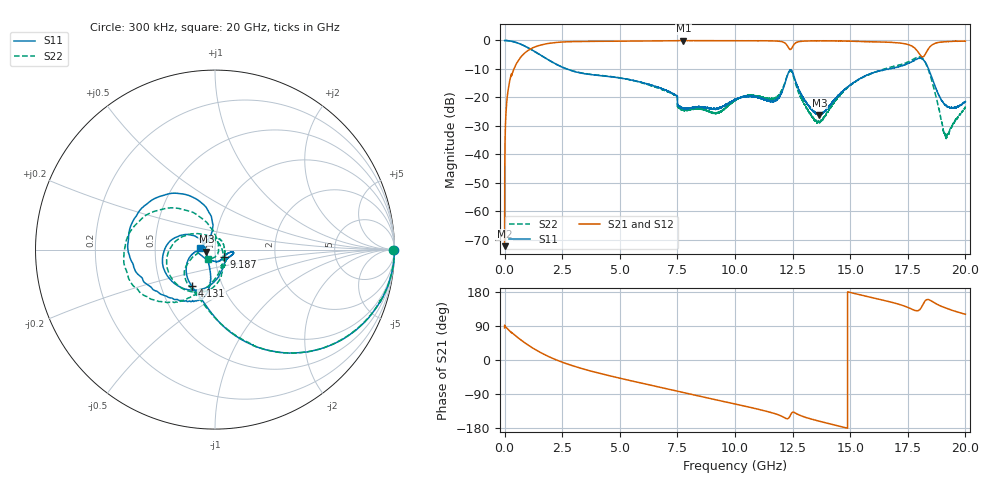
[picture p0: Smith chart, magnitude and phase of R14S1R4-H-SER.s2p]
!{R14S1R4}
!Johanson Technology Inc.
!www.johansontechnology.com
!Test Board Conditions:
!Substrate Type  RO4350B
!Substrate Thickness  20 mil
!Substrate Dk  3.66
!TL Type: GCPW
!TL Trace Width  36 mil
!TL Gap  12 mil
!Electrode orientation  Horizontal
!DUT TOPOLOGY	SERIES
!Mounting Pad LxW  26x36 mil
! Created Wed Nov 25 17:33:21 2020
! 2 Port Network Data from SP1.SP block
! freq  magS11  angS11  magS21  angS21  magS12  angS12  magS22  angS22
# khz S ma R 50
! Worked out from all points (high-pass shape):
!   20001 points, 300 kHz to 20 GHz, reference 50 ohm
!   highest |S21| = -0.05 dB at 7.757 GHz (marker M1); lowest = -72.2 dB at 300 kHz (marker M2)
!   |S21| within 3 dB of the highest: 1.111 GHz to 12.37 GHz (11.26 GHz wide, 167 % of centre); 12.43 GHz to 17.85 GHz (5.416 GHz wide, 35.8 % of centre)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
!   lowest |S11| = -26.2 dB at 13.66 GHz (marker M3), VSWR 1.10, Z = 45.4 - j1.11 ohm
!   |S11| at or under -10 dB: 2.693864 GHz to 2.696229 GHz (2.364 MHz wide, 0.0877 % of centre); 2.696 GHz to 16.69 GHz (13.99 GHz wide, 144 % of centre); 18.4 GHz to end of sweep
!   |S22| runs from -34.5 to 0.0 dB; largest |S21 - S12| = 0.016
!   S11 on the Smith chart (normalised r, x): 300 kHz: open; 4.131 GHz: 0.72, -0.31; 9.187 GHz: 1.10, -0.09; 20 GHz: 0.84, +0.02
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300  0.9954 -0.0  0.0002451 84.7  0.0002459 91.5  0.9943 -0.0
101300  0.9958 -6.2  0.09049 83.8  0.09079 83.7  0.9952 -6.1
134300  0.9925 -8.1  0.1195 81.7  0.12 81.8  0.9921 -8.0
513300  0.9174 -27.5  0.3911 62.2  0.3921 62.3  0.9164 -27.2
1785300  0.4875 -77.3  0.8689 12.7  0.87 12.7  0.4864 -77.1
3334300  0.2672 -110.6  0.9596 -22.3  0.9594 -22.2  0.2694 -113.4
4131300  0.2421 -122.1  0.9655 -35.3  0.9661 -35.3  0.2443 -127.9
6667300  0.1505 -162.1  0.9844 -70.9  0.9841 -70.9  0.146 -158.2
7757300  0.06526 -116.3  0.9941 -85.8  0.9928 -85.8  0.06087 125.4
9187300  0.06384 -37.7  0.9922 -105.2  0.9934 -105.3  0.05305 5.4
1.00003e7  0.09248 -8.4  0.9897 -116.1  0.9886 -116.1  0.08857 -50.5
1.17413e7  0.08722 -47.8  0.9777 -141.9  0.9773 -141.8  0.09867 -67.0
1.24063e7  0.3036 -153.1  0.6937 -145.4  0.699 -145.6  0.29 -146.5
1.33343e7  0.06166 162.4  0.9832 -156.3  0.983 -156.2  0.04572 75.4
1.36623e7  0.04918 -165.6  0.9833 -161.5  0.9844 -161.4  0.03754 20.6
1.50223e7  0.1682 -98.2  0.97 177.9  0.9715 177.7  0.1641 -90.8
1.66673e7  0.3115 -113.9  0.9312 154.3  0.9223 154.0  0.3339 -121.8
1.76473e7  0.4159 -150.5  0.8102 135.0  0.7989 134.7  0.4468 -141.5
1.81733e7  0.4576 146.6  0.5181 148.4  0.513 149.2  0.4687 164.0
1.85643e7  0.2106 99.3  0.8413 154.3  0.8395 154.5  0.1812 111.5
1.91493e7  0.07329 116.4  0.9547 136.9  0.9531 137.1  0.01984 4.2
2e7  0.0847 172.4  0.9719 120.7  0.9696 120.7  0.0674 -128.7
